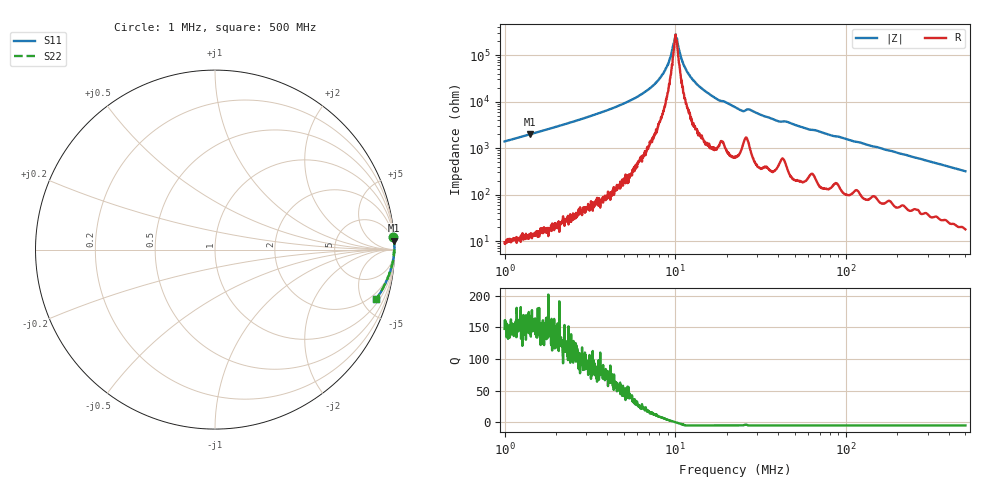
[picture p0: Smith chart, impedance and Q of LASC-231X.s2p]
!s-Parameter Generated by FASTRON Sdn. Bhd.
!FASTRON P/N : LASC-231X
!Keysight Technologies,E4991B,MY54100416,A.01.15
!Date: Tue Mar 17 15:51:06 2026
!Version  : Rev00 Tue Mar 17 15:51:06 2026
!Data & Calibration Information:
!PortZ  Port1:50+j0  Port2:50+j0
!When reading, reference impedance value at option line is always used.
!Remarks : This data is being provided solely for informational purposes.
!Freq	S11	S21	S12	S22
# Hz S dB R 50
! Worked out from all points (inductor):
!   1601 points, 1 MHz to 500 MHz, reference 50 ohm
!   read as one part in series: L = 219 uH near 1.032 MHz
!   highest Q = 161 at 1.407 MHz (marker M1), where L = 224 uH
!   self-resonance near 10.05 MHz
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1000000  -0.03 4.1  -22.90 -85.5  -22.90 -85.5  -0.03 4.1
1407484  -0.01 2.9  -25.93 -86.7  -25.93 -86.7  -0.01 2.9
2820919  -0.00 1.4  -32.53 -88.0  -32.53 -88.0  -0.00 1.4
5631849  -0.00 0.5  -41.06 -87.9  -41.06 -87.9  -0.00 0.5
6892354  -0.00 0.3  -45.06 -86.3  -45.06 -86.3  -0.00 0.3
7957584  -0.00 0.2  -49.34 -83.3  -49.34 -83.3  -0.00 0.2
8941017  -0.00 0.1  -55.18 -77.2  -55.18 -77.2  -0.00 0.1
9331304  -0.00 0.1  -58.75 -68.7  -58.75 -68.7  -0.00 0.1
9814575  -0.00 0.0  -65.20 -42.1  -65.20 -42.1  -0.00 0.0
1.004599e7  -0.00 0.0  -68.91 -0.4  -68.91 -0.4  -0.00 0.0
1.028286e7  -0.00 -0.0  -65.40 38.2  -65.40 38.2  -0.00 -0.0
1.081541e7  -0.00 -0.1  -58.97 69.7  -58.97 69.7  -0.00 -0.1
1.128751e7  -0.00 -0.1  -55.30 77.9  -55.30 77.9  -0.00 -0.1
1.293118e7  -0.00 -0.2  -48.73 83.6  -48.73 83.6  -0.00 -0.2
1.737158e7  -0.01 -0.5  -41.28 84.6  -41.28 84.6  -0.01 -0.5
2.236068e7  -0.01 -0.7  -37.66 84.4  -37.66 84.4  -0.01 -0.7
2.473679e7  -0.02 -0.9  -36.00 79.3  -36.00 79.3  -0.02 -0.9
2.72593e7  -0.02 -0.8  -36.56 80.4  -36.56 80.4  -0.02 -0.8
3.957791e7  -0.03 -1.5  -31.73 82.8  -31.73 82.8  -0.03 -1.5
6.307767e7  -0.05 -2.3  -27.93 81.2  -27.93 81.2  -0.05 -2.3
1.77937e8  -0.13 -6.3  -19.11 78.9  -19.11 78.9  -0.13 -6.3
5e8  -0.55 -17.2  -10.59 69.6  -10.59 69.6  -0.55 -17.2
